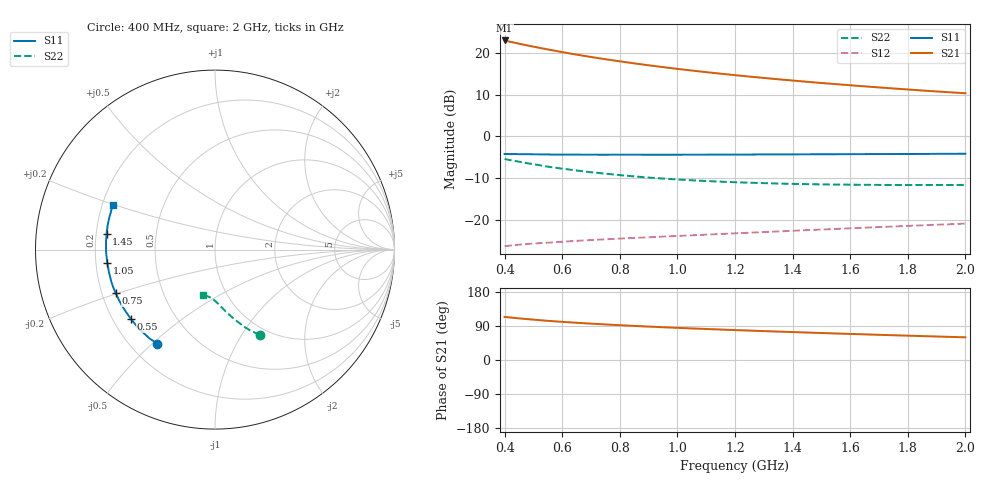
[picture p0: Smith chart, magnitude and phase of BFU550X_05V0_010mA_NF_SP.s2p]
! Filename:  P:\Prog\Test\Noise\ATS_data\Testdata_Net\BFU550X no attenuator noise\BFU550X_APG2013_44_C05_05p0V_010mA_NF_CM01_D.sf
! Date/Time: Fri 26/Jul/2013 14:37:12
! BFU550X_APG2013_44_C05_05p0V_1to10mA_NF_CM01_Bias5_R.sf
! Noise Parameter Data File
! BFU550X_APG2013_44_C05_05p0V_1to10mA_NF_CM01
! Date/time: Wed Jul 24 16:36:15 2013
! VAR V_out= 5.000000
! VAR I_out= 10.000000
! VAR V_in= 0.823500
! VAR I_in= 0.110610
! Device data file deembeded for feedlines and parallel
! Original file: \BFU550X no attenuator noise\BFU550X_APG2013_44_C05_05p0V_010mA_NF_CM01_R.sf
! Feed-files: PR005V01_100713_Feed1.s2p, PR005V01_100713_Feed2.s2p
! Parallel-file: PR005V01_100713_Par.s2p
# MHz S MA R 50
!  Freq-MHz  S11-mag  S11-arg  S21-mag  S21-arg  S12-mag  S12-arg  S22-mag  S22-arg
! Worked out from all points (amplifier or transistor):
!   37 points, 400 MHz to 2 GHz, reference 50 ohm
!   highest |S21| = 22.9 dB at 400 MHz (marker M1)
!   |S21| within 3 dB of that: start of sweep to 617.8 MHz
!   unconditionally stable (mu >= 1): 1.919 GHz to end of sweep
!   at 500 MHz: K = 0.43, MSG = 23.5 dB, |S12| = -25.6 dB
!   at 1.1 GHz: K = 0.78, MSG = 19.4 dB, |S12| = -23.5 dB
!   at 2 GHz: K = 1.01, MAG = 15.0 dB, |S12| = -20.8 dB
!   lowest NFmin = 0.78 dB at 440 MHz
!   S11 on the Smith chart (normalised r, x): 400 MHz: 0.31, -0.52; 550 MHz: 0.27, -0.34; 750 MHz: 0.26, -0.20; 1.05 GHz: 0.25, -0.06; 1.45 GHz: 0.24, +0.07; 2 GHz: 0.24, +0.20
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400  0.6166 -121.7  14.02 113.7  0.0487 43.1  0.5366 -62.5
420  0.6139 -124.4  13.5 112.1  0.04952 42.6  0.5192 -64.0
440  0.6141 -127.3  13.06 110.6  0.05037 42.0  0.5047 -65.1
460  0.6119 -129.8  12.61 109.2  0.05106 41.4  0.4916 -66.5
500  0.6104 -134.7  11.81 106.5  0.05239 40.4  0.4656 -68.8
550  0.6076 -140.4  10.96 103.3  0.05355 39.7  0.4346 -71.3
600  0.6055 -144.9  10.17 100.7  0.05508 39.2  0.4116 -73.6
650  0.6055 -149.2  9.492 98.2  0.05638 38.8  0.391 -75.6
700  0.6042 -153.0  8.892 95.9  0.05759 38.7  0.3729 -77.5
750  0.6039 -156.4  8.361 93.9  0.05883 38.6  0.3581 -79.1
800  0.6047 -159.7  7.892 91.8  0.06 38.6  0.3445 -80.8
850  0.6046 -162.7  7.466 90.0  0.06107 38.7  0.3325 -82.3
950  0.6039 -168.1  6.731 86.5  0.06337 39.1  0.3132 -85.0
1050  0.605 -172.8  6.127 83.3  0.06567 39.7  0.2986 -87.3
1100  0.6051 -175.0  5.861 81.8  0.0669 40.0  0.2926 -88.5
1200  0.6069 -179.1  5.396 79.0  0.06936 40.5  0.2831 -90.6
1300  0.6079 177.2  4.996 76.3  0.07185 41.1  0.2762 -92.5
1450  0.6103 172.0  4.495 72.4  0.07567 41.9  0.2687 -95.3
1500  0.6113 170.4  4.347 71.2  0.07695 42.2  0.2667 -96.2
1600  0.6132 167.3  4.085 68.8  0.07967 42.7  0.2646 -97.9
1750  0.6152 162.9  3.738 65.3  0.08367 43.3  0.2625 -100.4
2000  0.6208 156.3  3.276 59.9  0.09076 44.1  0.2632 -104.3
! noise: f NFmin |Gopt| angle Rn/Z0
400  0.8488  0.09871  154.2  0.082
460  0.8055  0.127  174.3  0.0727
600  0.8473  0.1133  164.3  0.0831
800  0.8445  0.177  166.9  0.0681
1000  0.8737  0.2096  171.9  0.0634
1200  0.9237  0.2512  172.6  0.0583
1400  0.9213  0.2718  178.2  0.0586
1600  0.9503  0.297  -178  0.0585
1800  0.9809  0.3275  -175  0.0563
2000  1.002  0.3558  -170.4  0.0563
